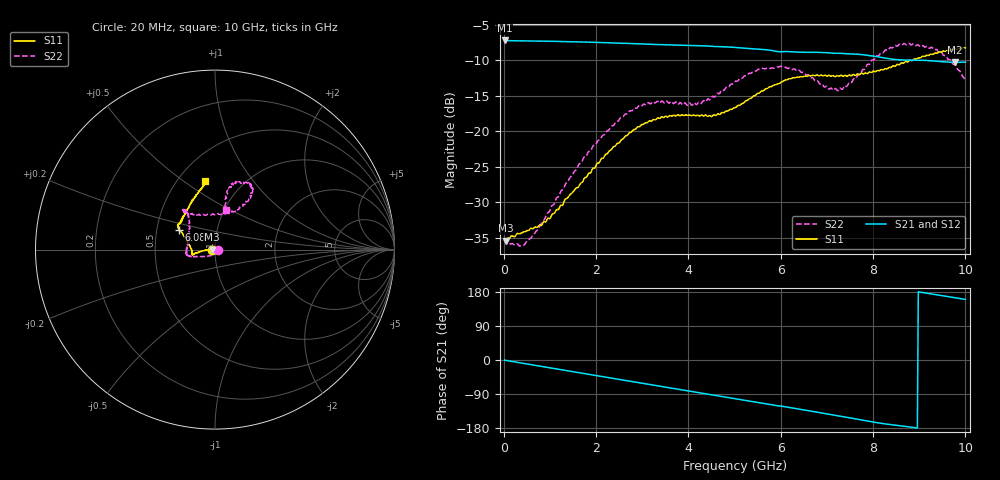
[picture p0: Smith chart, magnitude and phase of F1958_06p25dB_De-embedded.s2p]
! Integrated Device Technology
! Corporate Headquarters
! 6024 Silver Creek Valley Road
! San Jose, CA 95138  USA
! Phone:  1-408-284-8200
! Toll Free:  1-800-223-1366
! Webpage:  http://www.idt.com/
! Timing and RF Division
! 515 Groton Road, Suite 102
! Westford, MA 01886-6024
! Device:  F1958
! Description: 7-bit 0.25 dB Digital Step Attenuator
! Frequency:  0.001 -  6.000 GHz
! Package:  4x4 mm Thin QFN Plastic Package: 24 pin
! Ports:  2 RF, 12 DC
!  Pin  1  = D0
!  Pin  2  = VDD
!  Pin  3  = VMODE
!  Pin  4  = GND
!  Pin  5  = RF1  =  Port 1
!  Pin  6  = GND
!  Pin  7  = GND
!  Pin  8  = GND
!  Pin  9  = GND
!  Pin 10  = GND
!  Pin 11  = GND
!  Pin 12  = GND
!  Pin 13  = GND
!  Pin 14  = RF2  =  Port 2
!  Pin 15  = GND
!  Pin 16  = LE
!  Pin 17  = CLK
!  Pin 18  = DATA
!  Pin 19  = D6
!  Pin 20  = D5
!  Pin 21  = D4
!  Pin 22  = D3
!  Pin 23  = D2
!  Pin 24  = D1
! State:  25
! Atten State:  6.25 dB
! Voltage:  +3.30 Volts
! Current:  0.258 mA
! Data:  The device was measured on a F1958 evaluation board which has
!  individual transmission lines to the RF pins.  Data was collected
!  using a calibrated network analyzer.  The evaluation board was
!  de-embedded using Automatic Fixture Removal (AFR).
!  The reference plane is the edge of the package pin.
! Misc:
!  Action Tracker AT0419
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# GHz S dB R 50
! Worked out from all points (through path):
!   500 points, 20 MHz to 10 GHz, reference 50 ohm
!   highest |S21| = -7.19 dB at 20 MHz (marker M1); lowest = -10.3 dB at 9.78 GHz (marker M2)
!   group delay of S21, straight-line fit = 55.8 ps
!   lowest |S11| = -35.5 dB at 40 MHz (marker M3), VSWR 1.03, Z = 48.3 - j0.0894 ohm
!   |S11| at or under -10 dB: start of sweep to 8.793 GHz; 8.81068 GHz to 8.852684 GHz (42 MHz wide, 0.476 % of centre)
!   |S22| runs from -36.2 to -7.6 dB; largest |S21 - S12| = 0.0014
!   S11 on the Smith chart (normalised r, x): 20 MHz: 0.97, -0.00; 6.08 GHz: 0.65, +0.15; 10 GHz: 0.68, +0.61
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0.02  -35.41 -177.1  -7.19 -0.6  -7.19 -0.5  -35.12 -8.3
0.04  -35.45 -176.9  -7.20 -1.0  -7.20 -1.0  -35.38 -12.8
0.38  -34.37 174.0  -7.25 -8.0  -7.25 -7.9  -36.08 -46.1
0.56  -33.88 173.3  -7.27 -11.6  -7.26 -11.6  -35.23 -65.3
0.96  -32.25 177.7  -7.30 -19.8  -7.30 -19.8  -31.48 -100.9
1.7  -27.23 -175.9  -7.41 -34.9  -7.41 -34.9  -24.23 -143.0
2.58  -21.12 -170.4  -7.59 -52.8  -7.58 -52.9  -18.02 -162.0
2.92  -19.38 -169.1  -7.67 -59.7  -7.66 -59.8  -16.45 -166.4
3.36  -18.18 -167.6  -7.78 -68.6  -7.78 -68.7  -15.94 -171.0
4.24  -17.88 -171.8  -7.94 -86.4  -7.95 -86.4  -15.92 158.9
5.02  -16.67 168.8  -8.18 -102.3  -8.19 -102.3  -12.94 130.7
5.52  -14.64 157.4  -8.43 -112.5  -8.44 -112.5  -11.25 127.0
6.08  -12.84 151.1  -8.76 -123.0  -8.78 -123.0  -10.98 128.2
6.68  -12.13 146.7  -8.87 -135.1  -8.89 -135.0  -12.44 122.4
7.04  -12.11 143.6  -8.93 -143.1  -8.94 -143.0  -14.07 105.4
7.3  -12.11 141.6  -9.01 -148.4  -9.02 -148.3  -13.95 85.3
7.9  -11.74 130.8  -9.30 -161.5  -9.29 -161.5  -10.56 58.4
8.34  -11.02 121.1  -9.76 -169.9  -9.77 -170.0  -8.43 56.6
8.74  -10.24 112.6  -9.98 -175.9  -9.99 -175.8  -7.75 61.8
9.24  -9.15 102.8  -10.06 174.6  -10.06 174.6  -8.27 72.5
9.78  -8.38 98.1  -10.29 164.5  -10.31 164.5  -10.63 77.9
10  -8.24 97.9  -10.26 159.9  -10.29 160.0  -12.84 74.7
